FUNCTION_BLOCK FB 17
TITLE = FactoryLink S7 Send
// KNOW_HOW_PROTECT
AUTHOR : DLink
FAMILY : S7_H1
NAME   : S7_SEND
VERSION: 1.0


VAR_INPUT
  ACT         : BOOL;                  // Trigger to start a WRITE operation
  ID          : WORD;                  // Connection number, taken from CO configuration
  SEND        : ANY;                   // Data address
  LEN         : INT;                   // Number of words to transmit 1-112
END_VAR

VAR_OUTPUT
  DONE        : BOOL;                  // Set when a write cyclus is completed
  ERROR       : BOOL;                  // Errors: parameters, send and receive
  STATUS      : WORD;                  // Error code
END_VAR

VAR
  Send_Buf    : STRUCT                 // Buffer to send "Write" request to a partner
   Sys_ID     : WORD := W#16#5335;     // Must contain 'S5' chars
   Opcod1     : WORD := W#16#1001;     // Must contain the value b#(16,01)
   Opcod2     : WORD := W#16#303;      // Must contain the value b#(03,03)
   Opcod3     : WORD := W#16#308;      // Must contain the value b#(03,08)
   Org_ID     : BYTE;                  // Must contain the value 01 = DB request
   DB_No      : BYTE;                  // The target DB no. 1-255
   DW_No      : WORD;                  // The start offset = Start DW no. 0-2047
   Len        : WORD;                  // No of WORDs  1-112 are allowed for CP443/343
   End_blck   : WORD  := W#16#FF02;    // End header info. must contain B#(255,02)
   Data       : ARRAY [0..8192] OF BYTE;// Real data to the H1 partner
  END_STRUCT;
  Recv_Buf    : STRUCT                 // Receive buffer for a partners "Write" Reply
   Sys_ID     : WORD;                  // Must contain 'S5' chars
   Opcod1     : WORD;                  // Must contain the value b#(16,01)
   Opcod2     : WORD;                  // Must contain the value b#(03,04)
   Opcod3     : WORD;                  // Must contain the value b#(0f,03)
   Err_No     : BYTE;                  // Contains either 0 = OK or errorcode
   Emp_Blck   : BYTE;                  // Always xff, Indicating empty block
   Emp_Len    : BYTE;                  // Lenght of unused header info
   DispHead0  : BYTE;                  // Not used byte part of header
   DispHead1  : WORD;                  // Not used part of header
   DispHead2  : WORD;                  // Not used part of header
  END_STRUCT;
  R_NDR       : BOOL;                  // Set when data retrieved
  R_ERROR     : BOOL;                  // Set when there was an error by AG-RECV
  S_DONE      : BOOL;                  // Set when there AG-SEND completes a frame
  S_ERROR     : BOOL;                  // Set when AG-SEND has an error
  S_ACT       : BOOL;                  // Trigger to send a new frame with AG-SEND
  JOB_ACTIVE  : BOOL;                  // Indicates that a job is running
  WAIT_RECV   : BOOL;                  // Send data completed waiting for a Ackn. tlg
  EndTime     : TIME;                  // Calc. timeout point for a complete "write" cyclus
  R_LEN       : WORD;                  // No. of BYTES received
  S_LEN       : WORD;                  // No. of bytes to transmit to partner
  JOB_TIME_OUT: TIME := T#5S;          // completion timeout
  SFB_12    : SFB 12;                  // Local instance of SFB 12
  SFB_13    : SFB 13;                  // Local instance of SFB 13
END_VAR

VAR_TEMP
  Source_Ptr  : ANY;                   // Pointer to the target Data in this PLC's DB
  Dest_Ptr    : ANY;                   // Pointer to the internal data buf with user data
  Recv_Ptr    : ANY;                   // Pointer to the recv area in this instance DB
  Send_Ptr    : ANY;                   // Pointer to send area in this instance DB
  EN_STATUS   : BOOL;                  // Used only for EN, ENO operation
  TLG_ACKN_OK : BOOL;                  // Set when a acknowledge telegram is receieved from partner
  Sys_clock   : TIME;                  // Current PLC time
  Int_Var     : INT;                   // Temporary integer value
  Max_Adr     : DWORD;                 // Maximum source address
  Act_Adr     : INT;                   // Actual source address
  DB_Offset   : WORD;                  // DB Number offset for nr. > 255
  Adr_Offset  : WORD;                  // Address offset for nr. > 255
  LADDR       : DWORD;                 // CP module logical Baseaddress, from System Configuration
  S5          : BOOL;                  // S5 Addressing mode, when true
END_VAR


BEGIN
NETWORK
TITLE =

      SET   ;
      SAVE  ;
      =     #EN_STATUS;                // Save if any uses the EN, ENO status
      SET   ;                          // Make sure all info bits are zero
      R     #R_NDR;
      R     #S_DONE;
      R     #S_ACT;                    // Needed only as a oneshot
      R     #R_ERROR;
      R     #S_ERROR;
      R     #ERROR;
      R     #DONE;
      R     #S5;
      L     0;
      T     #STATUS;                   // Clear it, should only be set in one cycle
//
// Prepare the needed ANY pointers, so most of the initialization are done now.
// Cannot use static area for ANY pointers, must use local variable and build them up
//
      L     W#16#1002;                 // This is a type ANY BYTE Pointer = 02
      T     LW    10;                  // DestPtr
      T     LW    20;                  // Our local receivebuffer
      T     LW    30;                  // Our local send buffer
      L     8192;                      // Max len (Bytes)
      T     LW    12;                  // to Dest_Ptr (Data[0..223])
      L     16;                        // BYTE Lenght of receive buffer
      T     LW    22;                  // to Recv_ptr
      L     8192;                      // BYTE Lenght of send_buffer, only header
      T     LW    32;                  // to Send_Ptr
      L     DINO;                      // our own instance DB no
      T     LW    14;                  // Dest_Ptr is always in our own DB
      T     LW    24;                  // Recv_Ptr Too
      T     LW    34;                  // Same with Send_ptr
      L     W#16#8400;                 // DB area type pointer
      T     LW    16;                  // set dest ptr
      T     LW    26;                  // set recv ptr
      T     LW    36;                  // set send ptr
      L     8230;                      // start offset for recv_buf
      SLW   3;                         // adjust to a bit pointer
      T     LW    28;                  // set for recv_ptr
      L     8230;                      // start offset for recv_buf
      SRW   13;                         // adjust to a bit pointer
      T     LB    27;                  // set for recv_ptr
      L     20;                        // start offset send_ptr
      SLW   3;
      T     LW    38;                  // set for send_ptr

      L     DIW    4;                  // Get any pointer
      T     LW     0;                  // Type definition
      L     DIW    6;
      T     LW     2;                  // Max. length
      L     DIW    8;
      T     LW     4;                  // Db number
      L     DIW   10;
      T     LW     6;                  // Area type
      L     DIW   12;
      T     LW     8;                  // Start address offset
      SRW   3;
      T     #Act_Adr;

      L     LB     1;                  // Get boundary
      SRW   1;
      L     LW     2;
      *I    ;
      T     #Int_Var;                  // Got the length in bytes
      L     #LEN;
      >=I   ;
      JC    L_OK;
      L     0;                         // Max. length source < #LEN, give error
      T     #LEN;
L_OK: NOP   0;
//
// *** START A NEW "WRITE" JOB ON USER REQUEST ***
//
      A     #JOB_ACTIVE;
      AN    #WAIT_RECV;
      JC    NJOB;                      // Skip if no trigger or job allready running
      A     #WAIT_RECV;
      JC    NERR;                      // Waiting for reply...
//      BEU;
      ON    #ACT;
      JC    NTLG;                      // Nothing to do, just quit
      L     1;                         // Min no. of words
      L     #LEN;                      // Get wanted no. of bytes
      >I    ;                          // Zero or less ?
      JC    PERR;
      L     8192;                      // Max no, of bytes
      >I    ;                          // To many words ?
      JC    PERR;
//
// Evaluate source
//
      L     LB     6;                  // Get destination type
      L     7;
      AW;
      T     #Int_Var;                  // Clean destination type
      L     1;                         // 1 <= destination <= 4
      <I    ;
      JC    PERR;
      L     4;
      L     #Int_Var;
      <I    ;
      JC    PERR;
      L     2;
      >I    ;
      JC    D_FB;
      L     #LEN;
      T     #Send_Buf.Len;             // Set Len into the header
      L     L#+8191;                   // Max address IB, QB = 8191
      T     #Max_Adr;
      L     #Int_Var;
      L     1;
      >I    ;
      JC    D_QB;
      L     B#16#3;
      T     #Send_Buf.Org_ID;
      JU    D_OK;
D_QB: L     B#16#4;
      T     #Send_Buf.Org_ID;
      JU    D_OK;
D_FB: L     3;
      L     #Int_Var;
      <I    ;
      JC    D_DB;
      L     #LEN;
      T     #Send_Buf.Len;             // Set Len into the header
      L     L#+2047;                   // Max address FB = 2047
      T     #Max_Adr;
      L     B#16#2;
      T     #Send_Buf.Org_ID;
      JU    D_OK;
D_DB: L     L#+65534;                  // Max address DB = 65534
      T     #Max_Adr;
      L     #LEN;
      AN    S5;
      JC    S7_1;
      SRW   1;                         // Correct for word boundary
      T     #Send_Buf.Len;             // Set Len into the header
      L     #Act_Adr;
      SRW   1;
      T     #Act_Adr;
      L     #Send_Buf.Len;
S7_1: T     #Send_Buf.Len;             // Set Len into the header
      L     B#16#1;
      T     #Send_Buf.Org_ID;
      L     1;                         // min. target DB no.
      L     LW     4;
      >I    ;
      JC    PERR;
      L     4096;                      // Max. target DB no.
      >I    ;
      JC    PERR;
      L     LW     4;
      L     DINO;
      ==I   ;
      JC    PERR;
D_OK: L     0;                         // Min. DW no.
      L     LW     8;
      SRW   3;
      >I    ;
      JC    PERR;
      L     #Max_Adr;                  // Max. DW no.
      >D    ;
      JC    PERR;
      L     #LEN;
      L     16;
      +I    ;
      T     #S_LEN;
//
// Copy data from local DB to our own instance DB's Sendbuffer
//
      L     36;                        // Start offset for Dest_ptr = Data[0]
      SLW   3;
      T     LW    18;                  // Now set for Dest_Ptr
      CALL  SFC   20 (
             SRCBLK  := #Source_Ptr,
             RET_VAL := #Int_Var,
             DSTBLK  := #Dest_Ptr);    // Pointer into our own instance DB

      L     0;                         // Should be Zero if OK.
      L     #Int_Var;                  // Get result from the block move
      ==I   ;
      JC    CONT;                      // Ok Continue if every thing is fine
PERR: L     W#16#FFFD;                 // *** Errorcode MUST BE CHANGED ***
      T     #STATUS;
      S     #ERROR;
      JU    NTLG;
//
// Create the H1 Fetch header information
//
CONT: L     'S7';
      T     #Send_Buf.Sys_ID;
      L     W#16#1001;
      T     #Send_Buf.Opcod1;
      L     W#16#303;
      T     #Send_Buf.Opcod2;
      L     W#16#308;
      T     #Send_Buf.Opcod3;
      L     256;                       // Max. db number = 255
      L     LW     4;                  // Db number
      >I    ;
      JC    DBNO;                      // Check for db number >= 256
      L     256;
      /I    ;
      T     #DB_Offset;
      L     119;
      L     DB_Offset;
      +I    ;
      T     #Send_Buf.Org_ID;
      L     LW     4;                  // Db number
      L     256;
      MOD   ;
DBNO :T     #Send_Buf.DB_No;
      L     #Act_Adr;
      T     #Send_Buf.DW_No;
      L     W#16#FF02;
      T     #Send_Buf.End_blck;
      SET   ;
      S     #JOB_ACTIVE;               // Indicate job accepted
      =     #S_ACT;                    // Initiate the send function
NJOB: L     3;                         //Remote id
      T     #LADDR;
      CALL  SFB_12 (
            REQ    := #S_ACT,
            R      := FALSE,
            ID     := #ID,
            R_ID   := #LADDR,
            DONE   := #S_DONE,
            ERROR  := #S_ERROR,
            STATUS := #STATUS,
            SD_1   := #Send_Ptr,
            LEN    := #S_LEN);

//
// The send function returns with a unknown error kode H7000
// after completing a sendjob or when not doing anything
// For now we just shortcircuit this problem but it must be solved by Siemens
//
      L     #STATUS;                   // Get send status
      L     W#16#7000;                 // Not Know error status
      <>I   ;                          // skip if not unknown status
      JC    NERR;
      L     W#16#8181;                 // force default status
      T     #STATUS;                   // Into the status info
      A     #S_ERROR;                  // and clear the error indikation
      R     #S_ERROR;
//
// ************ JOB TIMEOUT SUPERVISION **************
// ************ USING THE BUILD IN CLOCK *****************
//
NERR: A     #S_DONE;                   // When data sendt to partner
      A     #JOB_ACTIVE;               // And we have a job running
      S     #WAIT_RECV;                // Start waiting on reply
      AN    #WAIT_RECV;
      ON    #JOB_ACTIVE;
      JC    NTLG;                      // skip if not waiting or no jobs
      CALL  SFC   64 (                 // get current PLC system time
             RET_VAL := #Sys_clock);

      AN    #S_DONE;
      JC    NLOA;                      // skip initial loading, if not just completed send
      L     #Sys_clock;                // Timeout point = current time + user defined timeout
      L     #JOB_TIME_OUT;             // no. of sec. before timeout
      +D    ;
      T     #EndTime;                  // this is our timeout setpoint
      JU    NOTI;                      // skip first time around
NLOA: L     #Sys_clock;                // current PLC time
      L     #EndTime;                  // calc. timeout point
      <=D   ;                          // calc. timeout setpoint reached ?
      JC    NOTI;                      // skip until timeout condition
      S     #ERROR;                    // then abort the job now.
      R     #JOB_ACTIVE;               // and clear current job
      L     W#16#FFFF;                 // Code for timeout condition
      T     #STATUS;                   // Inform user which error it was
//
// *********** RECEIVE RESPONSE FROM A PASSIVE PARTNER **********
//
NOTI: L     3;                         // Remote id
      T     #LADDR;
      CALL  SFB 13,db13 (
            EN_R   := TRUE,
            ID     := #ID,             // Connection ID from CO config.
            R_ID   := #LADDR,          // Module base adr. from System Config.
            NDR    := #R_NDR,          // Set if data received
            ERROR  := #R_ERROR,        // Set if there was an error
            STATUS := #STATUS,         // Receive status information
            RD_1   := #Recv_Ptr,       // Our newly build ANY pointer to our own DB
            LEN    := #R_LEN);         // No of databytes received

//
// Anything received ??
//

      AN    #R_NDR;                    // Do not test anything if nothing received
      ON    #JOB_ACTIVE;               // Or a reception, when we do not want it
      O     #R_ERROR;                  // or errors in AG-RECV function
      JC    NTLG;
      R     #JOB_ACTIVE;               // This job is ended regardless of success or not
      L     16;
      L     #R_LEN;                    // Received data lenght
      <>I   ;                          // is it exactly 16 bytes ?
      JC    RERR;                      // otherwise is not a header
      L     'S7';                      // This must be the in first 2 bytes
      L     #Recv_Buf.Sys_ID;
      <>I   ;
      JC    RERR;
      L     0;                         // Clear first part of header info for next frame
      T     #Recv_Buf.Sys_ID;
      L     W#16#1001;                 // must contain this value
      L     #Recv_Buf.Opcod1;
      <>I   ;
      JC    RERR;
      L     W#16#304;                  // and this
      L     #Recv_Buf.Opcod2;
      <>I   ;
      JC    RERR;
      L     W#16#F03;                  // and this
      L     #Recv_Buf.Opcod3;
      <>I   ;
      JC    RERR;
      L     W#16#FF;                   // and this
      L     #Recv_Buf.Emp_Blck;
      <>I   ;
      JC    RERR;
      L     W#16#7;                    // and this
      L     #Recv_Buf.Emp_Len;
      <>I   ;
      JC    RERR;
      L     0;
      L     #Recv_Buf.Err_No;          // Get the reply from the partner
      T     #STATUS;                   // send it out
      ==I   ;
      S     #DONE;                     // Job completed witout any error
      JC    NTLG;                      // Complete this job now
      S     #ERROR;                    // Set error indication
      JU    NTLG;                      // And complete the job
RERR: S     #ERROR;                    // *** Error in telegram header ***
      L     W#16#FFFE;                 // Recieved Header not valid opcode
      T     #STATUS;                   // Info to the user
//
// Final work before exit from this function
//
NTLG: A     #R_ERROR;                  // Any error ?
      O     #S_ERROR;
      O     #ERROR;
      O     #DONE;                     // or job finished
      R     #JOB_ACTIVE;               // Removes current job
      R     #WAIT_RECV;                // and any hanging bits
      O     #R_ERROR;                  // error indication on either AG-RECV or AG-SEND
      O     #S_ERROR;
      O     #ERROR;
      AN    #DONE;
      =     #ERROR;                    // are send out
      CLR   ;                          // restore the EN status to ENO
      A     #EN_STATUS;
      SAVE  ;
END_FUNCTION_BLOCK
